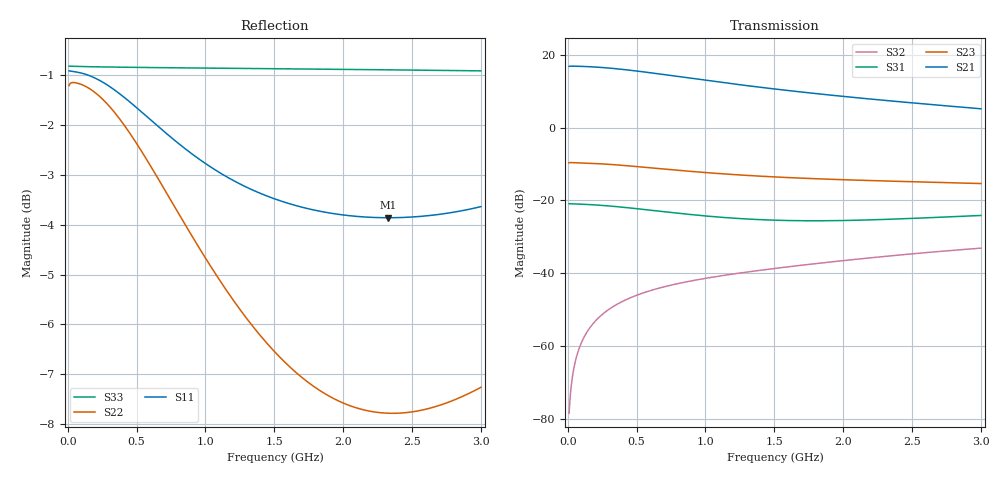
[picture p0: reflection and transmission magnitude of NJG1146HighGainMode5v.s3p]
! Created Mon Oct 18 18:39:42 2010
# hz S ma R 50
! 3 Port Network Data Port1:RFIN  Port2:RFOUT1  Port3:RFOUT2
! freq  magS11  angS11  magS12  angS12  magS13  angS13
!  magS21  angS21
!  magS22  angS22  magS23  angS23
!  magS31  angS31  magS32  angS32
!  magS33  angS33
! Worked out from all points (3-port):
!   2991 points, 10 MHz to 3 GHz, reference 50 ohm
!   strongest paths, dB at 10 MHz, 757 MHz, 1.505 GHz, 2.253 GHz, 3 GHz:
!     S21: 16.8, 14.2, 10.6, 7.6, 5.1
!     S23: -9.6, -11.6, -13.5, -14.6, -15.4
!     S31: -20.9, -23.3, -25.4, -25.2, -24.1
!     S32: -78.3, -43.1, -38.6, -35.5, -33.1
!   lowest |S11| = -3.9 dB at 2.329 GHz (marker M1), VSWR 4.57, Z = 12 - j15.4 ohm
!   |S11| at or under -10 dB: nowhere
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1e7  0.8993 -1.2  0.001909 57.5  0.09036 -0.4
     6.901 179.6  0.8695 -0.1  0.3296 179.8
     0.09035 -0.5  0.0001209 64.8  0.9091 -0.1
9.7e7  0.8949 -11.4  0.01581 79.9  0.0891 -2.9
       6.901 171.4  0.8718 -5.9  0.3272 174.2
       0.08898 -3.9  0.001099 83.4  0.9082 -0.8
3.09e8  0.8666 -35.2  0.04795 68.6  0.08547 -7.9
        6.512 153.0  0.8268 -18.3  0.3122 162.7
        0.08387 -10.5  0.003316 77.2  0.9073 -2.4
4.43e8  0.8388 -49.0  0.06526 61.1  0.08209 -10.2
        6.134 142.4  0.7818 -25.2  0.2983 156.3
        0.07934 -13.5  0.004539 74.2  0.9068 -3.4
5.84e8  0.8072 -62.2  0.08052 53.9  0.07829 -11.8
        5.69 132.3  0.7289 -31.3  0.2825 150.5
        0.07426 -15.6  0.005693 71.7  0.9063 -4.5
7.75e8  0.7665 -77.8  0.09687 45.5  0.0735 -12.8
        5.091 120.1  0.6579 -37.9  0.262 143.8
        0.06773 -16.8  0.007085 69.3  0.9057 -5.9
1.017e9  0.7237 -94.1  0.1122 37.0  0.0687 -12.5
         4.41 107.0  0.5791 -43.9  0.2402 137.0
         0.061 -15.9  0.008675 67.5  0.905 -7.7
1.505e9  0.6693 -118.5  0.1329 24.0  0.06343 -9.5
         3.374 85.4  0.4702 -50.1  0.2103 126.1
         0.0537 -9.5  0.01172 65.8  0.9038 -11.4
2.329e9  0.641 -144.0  0.1558 7.3  0.06323 -4.9
         2.332 56.1  0.4084 -53.1  0.1846 109.3
         0.05525 1.5  0.01731 62.5  0.9014 -17.5
3e9  0.6576 -157.4  0.1685 -6.4  0.06668 -5.0
     1.808 33.9  0.4336 -57.3  0.1707 93.9
     0.06231 3.2  0.02222 56.4  0.8994 -22.6
